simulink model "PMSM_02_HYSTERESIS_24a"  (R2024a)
settings: Solver=ode45  StartTime=0.0  StopTime=0.1  RelTol=1e-3  EnableMultiTasking=on
undefined symbols (not defined in the file): by, established, Flux, linkage, magnets, V
libraries: spsControlledVoltageSourceLib x3, spsCurrentMeasurementLib x3, spsPermanentMagnetSynchronousMachineLib x1, spspowerguiLib x1

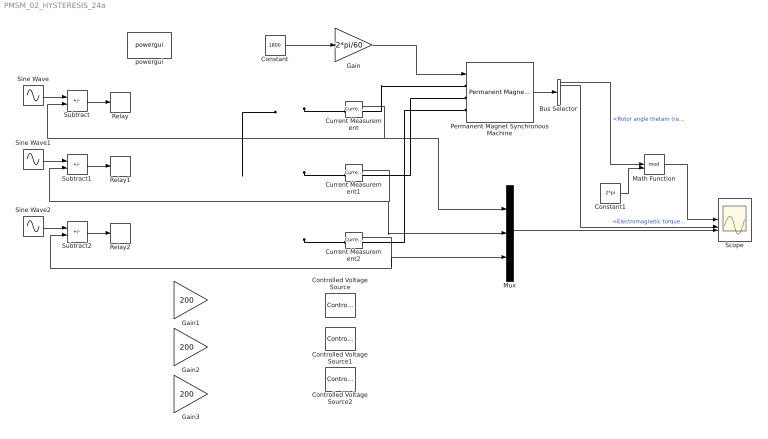
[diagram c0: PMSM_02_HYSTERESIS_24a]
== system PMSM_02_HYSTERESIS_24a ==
  Bus Selector : BusSelector  OutputSignals=Rotor angle thetam (rad),Electromagnetic torque Te (N*m)
  Constant : Constant  Value=1800
  Constant1 : Constant  Value=2*pi
  Controlled Voltage Source : spsControlledVoltageSourceLib/Controlled Voltage Source  Initialize=on  Source_Type=AC  Amplitude=0  Phase=0  Frequency=0  Measurements=None
  Controlled Voltage Source1 : spsControlledVoltageSourceLib/Controlled Voltage Source  Initialize=on  Source_Type=AC  Amplitude=0  Phase=0  Frequency=0  Measurements=None
  Controlled Voltage Source2 : spsControlledVoltageSourceLib/Controlled Voltage Source  Initialize=on  Source_Type=AC  Amplitude=0  Phase=0  Frequency=0  Measurements=None
  Current Measurement : spsCurrentMeasurementLib/Current Measurement  PhasorSimulation=off  OutputType=Complex  PSBequivalent=0
  Current Measurement1 : spsCurrentMeasurementLib/Current Measurement  PhasorSimulation=off  OutputType=Complex  PSBequivalent=0
  Current Measurement2 : spsCurrentMeasurementLib/Current Measurement  PhasorSimulation=off  OutputType=Complex  PSBequivalent=0
  Gain : Gain  Gain=2*pi/60
  Gain1 : Gain  Gain=200
  Gain2 : Gain  Gain=200
  Gain3 : Gain  Gain=200
  Math Function : Math  Operator=mod  SignedPower=on
  Mux : Mux  Inputs=3
  Permanent Magnet Synchronous Machine : spsPermanentMagnetSynchronousMachineLib/Permanent Magnet Synchronous Machine  NbPhases=3  FluxDistribution=Sinusoidal  RotorType=Round  MechanicalLoad=Speed w  PresetModel=No  ShowDetailedParameters=on  MeasurementBus=off  Resistance=0.423  Inductance=8.5e-3  dqInductances=[8.5e-3,8.5e-3]  La=0.00476  MachineConstant=Flux linkage established by magnets (V.s)  Flux=0.422  VoltageCst=153.0847  TorqueCst=1.266  Flat=120  Mechanical=[0.03 0.04 4 0]  PolePairs=2  InitialConditions=[0,0, 0,0]  InitialConditions5ph=[0 0 0 0 0 0]  RefAngle=Aligned with phase A axis (original Park)  IterativeDiscreteModel=Trapezoidal non iterative  TsBlock=-1  TsPowergui=0
  Relay : Relay  OnSwitchValue=0.1  OffSwitchValue=-0.1  OffOutputValue=-1
  Relay1 : Relay  OnSwitchValue=0.1  OffSwitchValue=-0.1  OffOutputValue=-1
  Relay2 : Relay  OnSwitchValue=0.1  OffSwitchValue=-0.1  OffOutputValue=-1
  Scope : Scope  NumInputPorts=3
  Sine Wave : Sin  Amplitude=-3  Frequency=2*pi*60  SampleTime=0
  Sine Wave1 : Sin  Amplitude=-3  Frequency=2*pi*60  Phase=-2*pi/3  SampleTime=0
  Sine Wave2 : Sin  Amplitude=-3  Frequency=2*pi*60  Phase=2*pi/3  SampleTime=0
  Subtract : Sum  Inputs=+-
  Subtract1 : Sum  Inputs=+-
  Subtract2 : Sum  Inputs=+-
  powergui : spspowerguiLib/powergui  Priority=1  SimulationMode=Continuous  SampleTime=50e-6  frequency=60  Iterations=50  frequencyindice=0  Pbase=100e6  ErrMax=1e-4  UnitsV=kV  UnitsW=MW  buscounter=0  FunctionMessages=off  echomessages=off  EnableUseOfTLC=off  CurrentSourceSwitches=off  DisableSnubberDevices=on  DisableRonSwitches=on  DisableVfSwitches=on  DisplayEquations=off  AutomaticDiscreteSolvers=off  SolverType=Tustin  Interpol=off  ExternalGateDelay=off  methode=off  Ts=0  x0status=blocks  SPID=on  SwTol=0  HookPort=off  NonlinearTolerance=1e-4  nMaxIteration=100  ContinueOnMaxIteration=off  RestoreLinks=warning  ResistiveCurrentMeasurement=off  Frange=[0:2:500]  Ylog=off  Xlog=on  ShowGrid=off  save=off  variable=ZData  structure=0  ZoomFFT=off  StartTime=0.0  cycles=1  DisplayStyle=1  fundamental=60  FreqAxis=off  MaxFrequency=1000  frequencyindicesteady=1  RmsSteady=1  display=off
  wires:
  Gain/1 -> Permanent Magnet Synchronous Machine/1
  Constant/1 -> Gain/1
  Current Measurement/1 -> Subtract/2, Mux/1
  Current Measurement1/1 -> Mux/2, Subtract1/2
  Current Measurement2/1 -> Mux/3, Subtract2/2
  Relay/1 -> ?
  Relay1/1 -> ?
  Relay2/1 -> ?
  ? -> ?
  ? -> ?
  ? -> ?
  Sine Wave/1 -> Subtract/1
  Subtract/1 -> Relay/1
  Subtract1/1 -> Relay1/1
  Sine Wave1/1 -> Subtract1/1
  Subtract2/1 -> Relay2/1
  Sine Wave2/1 -> Subtract2/1
  Permanent Magnet Synchronous Machine/1 -> Bus Selector/1
  Mux/1 -> Scope/3
  Bus Selector/2 -> Scope/2  "<Electromagnetic torque Te (N*m)>"
  Bus Selector/1 -> Math Function/1  "<Rotor angle thetam (rad)>"
  Math Function/1 -> Scope/1
  Constant1/1 -> Math Function/2
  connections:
  Current Measurement/RConn1 -- Permanent Magnet Synchronous Machine/LConn1
  Permanent Magnet Synchronous Machine/LConn2 -- Current Measurement1/RConn1
  Current Measurement2/RConn1 -- Permanent Magnet Synchronous Machine/LConn3
  Current Measurement2/LConn1 -- ?
  Current Measurement1/LConn1 -- ?
  Current Measurement/LConn1 -- ?
  ?
